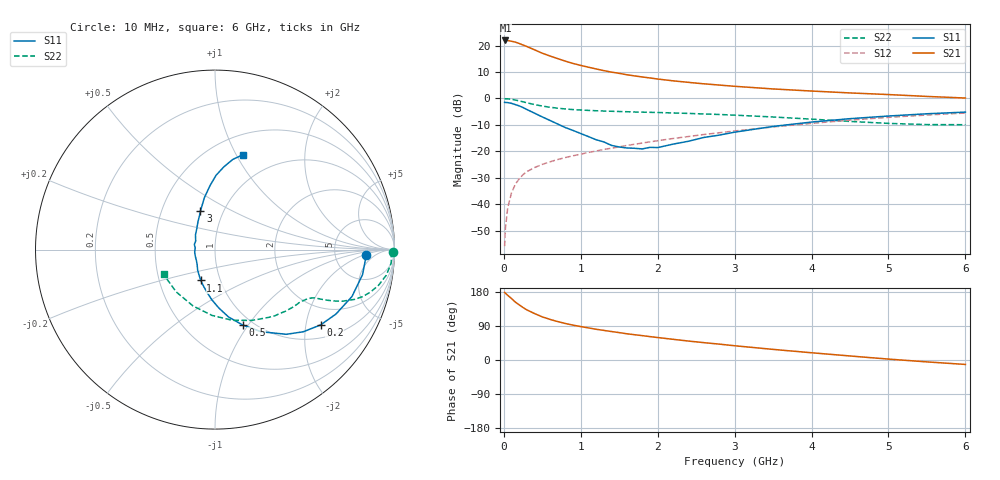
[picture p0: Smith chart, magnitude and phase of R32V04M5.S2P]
! SIEMENS Small Signal Semiconductors
! BFR181
! Si NPN RF Bipolar Junction Transistor in SOT23
! VCE = 2 V  IC = 4.5 mA
! Common Emitter S-Parameters:  May  1996
# GHz  S  MA  R  50
!  f  S11  S21  S12  S22
! GHz  MAG  ANG  MAG  ANG  MAG  ANG  MAG  ANG
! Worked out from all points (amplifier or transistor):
!   36 points, 10 MHz to 6 GHz, reference 50 ohm
!   highest |S21| = 21.9 dB at 20 MHz (marker M1)
!   |S21| within 3 dB of that: start of sweep to 355.9 MHz
!   unconditionally stable (mu >= 1): 1.134 GHz to 3.001 GHz
!   at 250 MHz: K = 0.39, MSG = 24.5 dB, |S12| = -28.8 dB
!   at 1.4 GHz: K = 1.05, MAG = 13.0 dB, |S12| = -18.8 dB
!   at 6 GHz: K = 0.86, MSG = 2.8 dB, |S12| = -5.5 dB
!   S11 on the Smith chart (normalised r, x): 10 MHz: 11, -2; 200 MHz: 1.38, -2.43; 500 MHz: 0.90, -0.94; 1.1 GHz: 0.81, -0.29; 3 GHz: 0.78, +0.35; 6 GHz: 0.70, +1.07
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0.01  0.8428 -2.0  12.44 178.2  0.0016 91.6  0.9936 -0.9
0.02  0.84 -3.8  12.51 176.1  0.0034 86.6  0.9828 -1.7
0.05  0.8339 -9.6  12.46 170.8  0.0085 86.2  0.9844 -4.4
0.1  0.8067 -18.9  12.06 162.1  0.0164 79.7  0.965 -8.5
0.15  0.7639 -28.0  11.63 152.6  0.0238 75.0  0.9328 -12.3
0.2  0.7228 -35.5  10.96 145.5  0.0301 72.0  0.8978 -15.3
0.25  0.6716 -43.0  10.25 138.4  0.0362 69.2  0.8625 -17.7
0.3  0.6168 -49.9  9.597 132.1  0.0413 67.0  0.8263 -19.6
0.4  0.5249 -60.7  8.31 122.5  0.0492 63.6  0.7647 -22.1
0.5  0.4469 -69.9  7.163 113.8  0.0565 62.3  0.7172 -23.5
0.6  0.3831 -78.6  6.355 107.2  0.0632 61.8  0.6812 -24.4
0.7  0.3277 -86.0  5.666 101.4  0.0697 62.1  0.6536 -25.0
0.8  0.2809 -93.5  5.071 96.3  0.0761 61.6  0.6322 -25.5
1.1  0.1896 -114.8  3.897 84.7  0.0951 62.5  0.5934 -27.2
1.3  0.1504 -129.9  3.359 78.1  0.1084 63.0  0.5778 -28.7
1.6  0.1155 -162.6  2.807 69.2  0.1289 63.1  0.5603 -31.4
2.2  0.1365 142.8  2.153 54.6  0.1745 62.0  0.531 -38.5
3  0.23 110.6  1.697 37.6  0.242 57.6  0.4826 -51.4
3.5  0.2951 101.6  1.512 28.0  0.2883 53.7  0.4455 -62.3
4.5  0.414 89.2  1.271 10.6  0.3879 43.4  0.3671 -92.6
5.5  0.5125 78.8  1.091 -5.0  0.4858 30.6  0.3198 -132.5
6  0.5511 73.6  1.018 -11.7  0.5292 23.4  0.3183 -154.2
